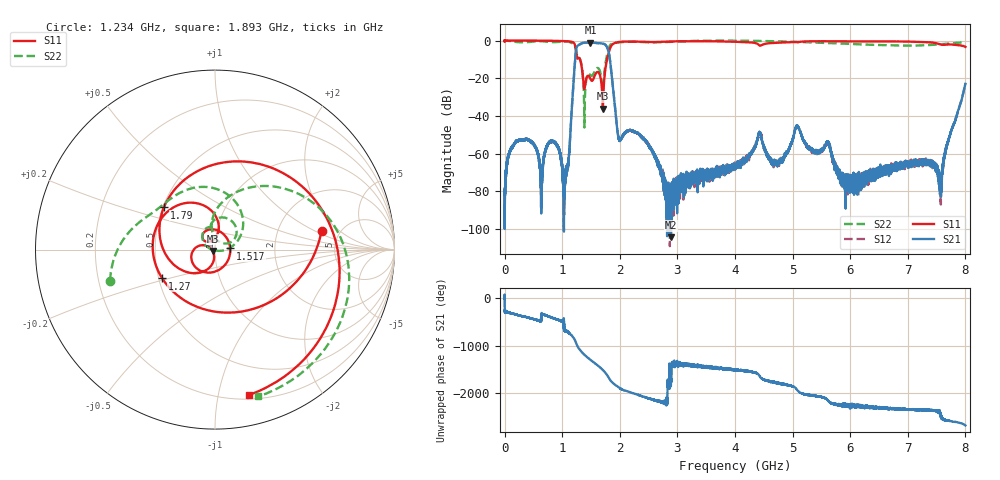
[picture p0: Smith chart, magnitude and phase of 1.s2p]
!Keysight Technologies,N5232A,MY52221221,A.10.65.11
!Date: Friday, October 20, 2023 10:51:06
!Correction: S11(Full 2 Port(1,4))
!S41(Full 2 Port(1,4))
!S14(Full 2 Port(1,4))
!S44(Full 2 Port(1,4))
!S2P File: Measurements: S11, S41, S14, S44:
# Hz S  RI  R 50
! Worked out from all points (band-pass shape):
!   16001 points, 300 kHz to 8 GHz, reference 50 ohm
!   highest |S21| = -1.15 dB at 1.491 GHz (marker M1); lowest = -104.4 dB at 2.884 GHz (marker M2)
!   |S21| within 3 dB of the highest: 1.247 GHz to 1.788 GHz (541.4 MHz wide, 35.7 % of centre)
!   lowest |S11| = -36.1 dB at 1.706 GHz (marker M3), VSWR 1.03, Z = 48.7 - j0.813 ohm
!   |S11| at or under -10 dB: 1.309 GHz to 1.78 GHz (471.2 MHz wide, 30.5 % of centre)
!   |S22| runs from -46.2 to 0.0 dB; largest |S21 - S12| = 0.0099
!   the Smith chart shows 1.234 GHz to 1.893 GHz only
!   S11 on the Smith chart (normalised r, x): 1.234 GHz: 3.62, +1.18; 1.27 GHz: 0.52, -0.19; 1.517 GHz: 1.19, +0.02; 1.79 GHz: 0.51, +0.28; 1.893 GHz: 0.23, -1.23
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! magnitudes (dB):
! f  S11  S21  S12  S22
! 300 kHz  0.0  -78.6  -88.5  0.0
! 348.8 MHz  0.0  -52.5  -52.6  -0.9
! 636.8 MHz  -0.1  -81.4  -79.9  -0.4
! 875.8 MHz  -0.2  -54.4  -54.6  -0.8
! 1.05 GHz  -0.3  -73.1  -73.9  -0.6
! 1.234 GHz  -4.4  -6.8  -6.9  -4.3
! 1.27 GHz  -9.5  -2.7  -2.6  -8.4
! 1.334 GHz  -13.1  -1.6  -1.6  -12.6
! 1.491 GHz  -20.4  -1.1  -1.2  -18.4
! 1.517 GHz  -21.4  -1.2  -1.2  -18.7
! 1.706 GHz  -36.1  -1.6  -1.6  -26.1
! 1.79 GHz  -8.7  -4.3  -4.4  -6.1
! 1.893 GHz  -1.6  -27.9  -28.0  -1.4
! 1.998 GHz  -0.7  -53.2  -52.7  -1.0
! 2.667 GHz  -0.7  -67.0  -64.7  -1.0
! 2.884 GHz  -0.5  -104.4  -79.0  -0.7
! 4 GHz  -0.7  -67.3  -67.6  -0.1
! 4.424 GHz  -2.6  -48.5  -49.4  -0.2
! 5.334 GHz  -0.4  -57.8  -58.9  -1.0
! 6.667 GHz  -0.5  -66.1  -67.4  -2.6
! 7.562 GHz  -2.1  -77.7  -78.1  -2.0
! 8 GHz  -3.4  -23.0  -22.6  -1.4
